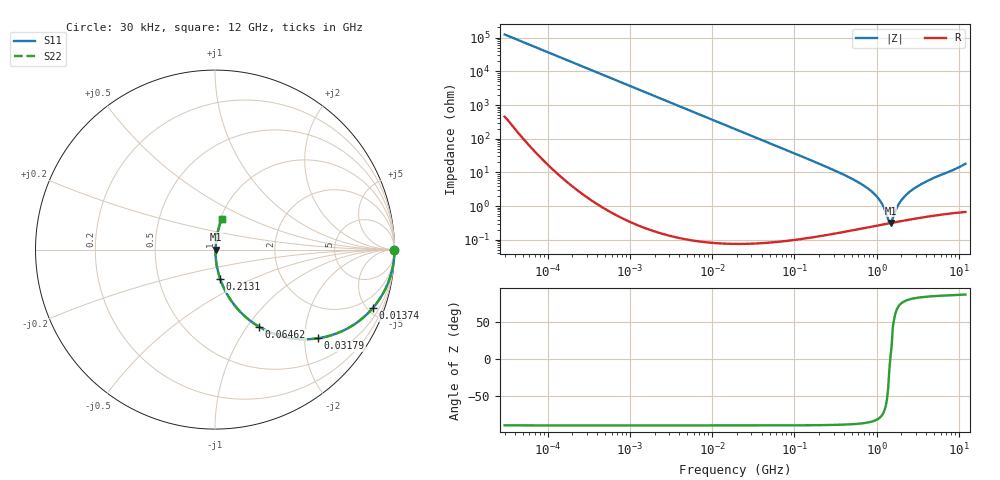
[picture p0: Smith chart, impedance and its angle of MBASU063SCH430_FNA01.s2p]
! MBASU063SCH430_FNA01  S-PARAMETER MODEL  ( General Type )
! Model Generated by TAIYO YUDEN Corporation (http://www.ty-top.com)
! Version 2.0
! TAIYO YUDEN Control No. 141022
! Copyright(c) 2013 TAIYO YUDEN CO.,LTD. All Rights Reserved.
! Product Description (link to TY-COMPAS)
! https://ds.yuden.co.jp/TYCOMPAS/or/detail?pn=MBASU063SCH430JFNA01&u=M
! Products Name : Multilayer Ceramic Capacitors
! Characteristics :
!  Capacitance : 43 pF , Rated Voltage : 50V , TCC : CH / C0H
!  Case Size : 0.6 x 0.3 / 0.024 x 0.012 [mm/inch] , Thickness : 0.3 / 0.012 [mm/inch]
!  (Conditions: Temperature = 25 degC , DC Bias Current/Voltage = 0A / 0V)
! External Node Assignments :
!  1  o---| |---o  2
! GND o---------o GND
! Frequency Range : 0.03MHz  -  12000MHz  [ 401 STEP ]
# MHz S RI R 50
! Freq[MHz].  S11 Real  S11 Imag  S21 Real  S21 Imag  S12 Real  S12 Imag  S22 Real  S22 Imag
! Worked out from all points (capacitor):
!   401 points, 30 kHz to 12 GHz, reference 50 ohm
!   read as one part in series: C = 43 pF near 32 kHz
!   lowest |Z| = 317 mohm at 1.475 GHz (marker M1)
!   series resonance near 1.465 GHz, so ESL is about 270 pH
!   S11 on the Smith chart (normalised r, x): 30 kHz: open; 13.74 MHz: 1.00, -5.39; 31.79 MHz: 1.00, -2.33; 64.62 MHz: 1.00, -1.14; 213.1 MHz: 1.00, -0.34; 12 GHz: 1.01, +0.36
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0.03  1 -0.000811  3.62e-06 0.000811  3.62e-06 0.000811  1 -0.000811
0.260295  0.9999 -0.00703  5.06e-05 0.00703  5.06e-05 0.00703  0.9999 -0.00703
2.258455  0.9963 -0.0608  0.00372 0.0608  0.00372 0.0608  0.9963 -0.0608
5.942454  0.9748 -0.1565  0.0252 0.1565  0.0252 0.1565  0.9748 -0.1565
13.74358  0.8787 -0.3263  0.1213 0.3263  0.1213 0.3263  0.8787 -0.3263
18.97367  0.7918 -0.4059  0.2082 0.4059  0.2082 0.4059  0.7918 -0.4059
31.78584  0.5753 -0.494  0.4247 0.494  0.4247 0.494  0.5753 -0.494
64.61702  0.2466 -0.4303  0.7534 0.4303  0.7534 0.4303  0.2466 -0.4303
98.2684  0.1239 -0.3281  0.8761 0.3281  0.8761 0.3281  0.1239 -0.3281
164.6252  0.048 -0.211  0.952 0.211  0.952 0.211  0.048 -0.211
213.0775  0.0293 -0.1648  0.9707 0.1648  0.9707 0.1648  0.0293 -0.1648
508.9517  0.00595 -0.0633  0.9941 0.0633  0.9941 0.0633  0.00595 -0.0633
852.6267  0.00324 -0.0283  0.9968 0.0283  0.9968 0.0283  0.00324 -0.0283
1139.739  0.00295 -0.0124  0.9971 0.0124  0.9971 0.0124  0.00295 -0.0124
1428.372  0.0031 -0.000754  0.9969 0.000754  0.9969 0.000754  0.0031 -0.000754
1475.185  0.00315 0.000214  0.9969 -0.000214  0.9969 -0.000214  0.00315 0.000214
1573.464  0.00325 0.00307  0.9967 -0.00307  0.9967 -0.00307  0.00325 0.00307
1790.1  0.00352 0.00901  0.9965 -0.00901  0.9965 -0.00901  0.00352 0.00901
1971.936  0.00378 0.0138  0.9962 -0.0138  0.9962 -0.0138  0.00378 0.0138
2635.962  0.00488 0.0285  0.9951 -0.0285  0.9951 -0.0285  0.00488 0.0285
4415.924  0.00855 0.0595  0.9914 -0.0595  0.9914 -0.0595  0.00855 0.0595
12000  0.0375 0.1722  0.9625 -0.1722  0.9625 -0.1722  0.0375 0.1722
